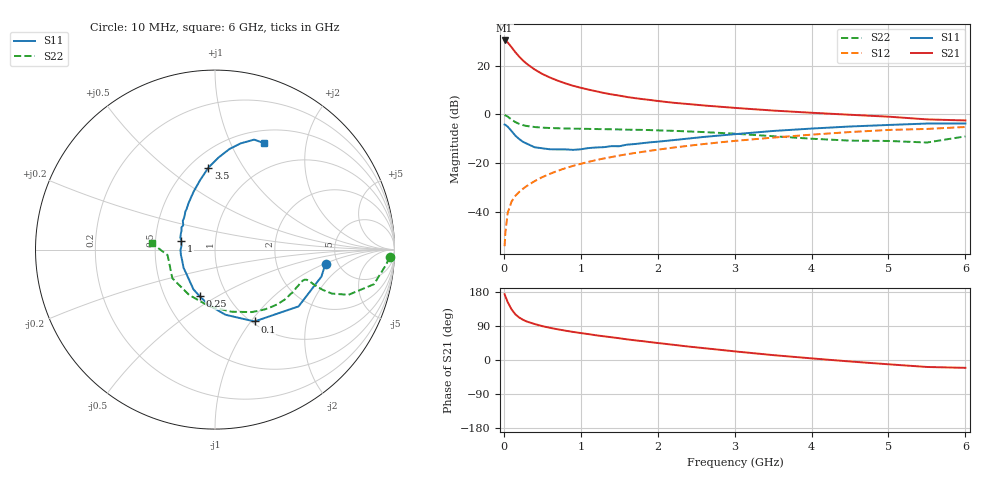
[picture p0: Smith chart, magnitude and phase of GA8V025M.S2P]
! Infineon Technologies  Discrete & RF Semiconductors
! BF775
! Si NPN RF Bipolar Junction Transistor in SOT23
! VCE = 8 V  IC = 25 mA
! Common Emitter S-Parameters:  May  1996
# GHz  S  MA  R  50
!  f  S11  S21  S12  S22
! GHz  MAG  ANG  MAG  ANG  MAG  ANG  MAG  ANG
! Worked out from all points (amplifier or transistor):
!   36 points, 10 MHz to 6 GHz, reference 50 ohm
!   highest |S21| = 30.3 dB at 10 MHz (marker M1)
!   |S21| within 3 dB of that: start of sweep to 105.7 MHz
!   unconditionally stable (mu >= 1): 384.6 MHz to 2.609 GHz
!   at 250 MHz: K = 0.87, MSG = 26.2 dB, |S12| = -30.4 dB
!   at 1.4 GHz: K = 1.10, MAG = 10.9 dB, |S12| = -17.5 dB
!   at 6 GHz: K = 0.90, MSG = 1.3 dB, |S12| = -5.1 dB
!   S11 on the Smith chart (normalised r, x): 10 MHz: 4.00, -1.01; 100 MHz: 1.03, -1.04; 250 MHz: 0.74, -0.42; 1 GHz: 0.68, +0.07; 3.5 GHz: 0.62, +0.71; 6 GHz: 0.65, +1.35
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0.01  0.6206 -7.2  32.8 173.8  0.002 83.7  0.9751 -2.5
0.02  0.6118 -14.2  32.28 168.1  0.0038 85.0  0.955 -5.3
0.05  0.5629 -34.2  29.89 152.9  0.0096 77.2  0.9061 -12.3
0.1  0.4569 -61.2  23.86 133.7  0.0164 69.7  0.7854 -18.7
0.15  0.3675 -80.9  18.81 120.4  0.0215 66.5  0.6967 -20.6
0.2  0.3131 -95.7  15.27 112.1  0.0258 67.3  0.6405 -20.5
0.25  0.2739 -108.1  12.69 106.0  0.0301 67.7  0.6029 -19.9
0.3  0.2516 -118.6  10.84 101.4  0.0344 68.7  0.5794 -19.3
0.4  0.2127 -136.5  8.355 95.0  0.043 70.4  0.5524 -18.4
0.5  0.2024 -150.0  6.749 89.3  0.052 71.3  0.5364 -18.2
0.6  0.1932 -160.5  5.703 85.0  0.0608 71.4  0.5276 -18.5
0.7  0.1922 -170.8  4.927 81.0  0.07 71.8  0.5211 -19.1
0.8  0.1924 -179.0  4.329 77.4  0.0792 71.3  0.5161 -20.0
1  0.1933 166.1  3.517 71.1  0.0973 70.9  0.5094 -21.9
1.1  0.2046 160.7  3.227 68.3  0.1068 70.3  0.5056 -23.4
1.3  0.2136 151.0  2.756 62.6  0.1252 69.0  0.4989 -25.9
1.6  0.2403 138.3  2.279 54.5  0.1531 66.6  0.4879 -30.6
2.2  0.2973 119.8  1.738 40.2  0.209 61.3  0.4618 -41.3
3.5  0.4584 94.6  1.201 12.9  0.3354 47.1  0.3582 -75.1
4.5  0.5663 81.8  0.985 -3.9  0.4358 34.1  0.2908 -119.8
5.5  0.6505 70.4  0.792 -18.4  0.5049 18.1  0.266 -173.3
6  0.6531 65.2  0.753 -20.7  0.5534 13.7  0.3555 174.1
